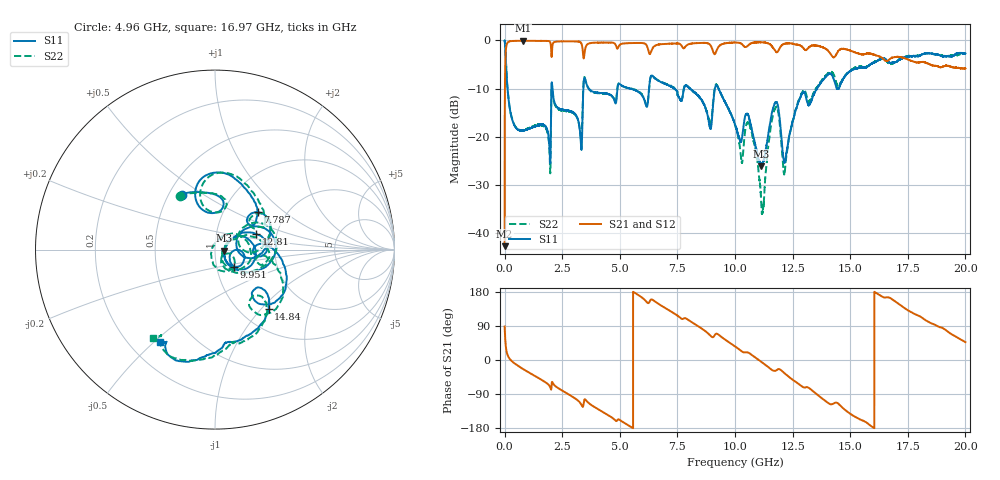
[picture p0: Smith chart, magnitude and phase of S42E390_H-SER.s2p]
! Created Wed Nov 25 22:14:23 2020
# khz S ma R 50
! 2 Port Network Data from SP1.SP block
! freq  magS11  angS11  magS21  angS21  magS12  angS12  magS22  angS22
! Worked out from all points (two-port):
!   20001 points, 300 kHz to 20 GHz, reference 50 ohm
!   highest |S21| = -0.07 dB at 794.3 MHz (marker M1); lowest = -42.8 dB at 300 kHz (marker M2)
!   |S21| within 3 dB of the highest: 40.74 MHz to 2.031 GHz (1.99 GHz wide, 192 % of centre); 3.459 GHz to 14.18 GHz (10.72 GHz wide, 122 % of centre)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
!   lowest |S11| = -26.2 dB at 11.15 GHz (marker M3), VSWR 1.10, Z = 55.1 - j0.678 ohm
!   |S11| at or under -10 dB: 126.5 MHz to 2.034 GHz (1.907 GHz wide, 177 % of centre); 2.075 GHz to 3.418 GHz (1.343 GHz wide, 48.9 % of centre); 9.28 GHz to 13.56 GHz (4.277 GHz wide, 37.5 % of centre)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
!   |S22| runs from -36.1 to 0.0 dB; largest |S21 - S12| = 0.016
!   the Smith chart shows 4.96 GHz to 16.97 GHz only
!   S11 on the Smith chart (normalised r, x): 4.96 GHz: 0.59, +0.41; 7.787 GHz: 1.44, +0.67; 9.951 GHz: 1.21, -0.24; 12.81 GHz: 1.57, +0.28; 14.84 GHz: 1.34, -1.10; 16.97 GHz: 0.33, -0.52
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300  0.9948 -0.3  0.007248 88.5  0.007244 89.5  0.993 -0.4
123300  0.3234 -75.8  0.9455 14.2  0.9454 14.2  0.3244 -75.9
794300  0.1155 -114.1  0.9918 -23.6  0.9902 -23.5  0.1168 -115.0
1911300  0.09897 -147.4  0.985 -65.4  0.9852 -65.4  0.094 -154.5
2121300  0.2507 -148.7  0.9472 -64.0  0.9477 -63.9  0.2455 -150.9
3334300  0.07255 -163.9  0.9276 -118.1  0.9282 -118.1  0.09135 -149.6
3512300  0.3819 173.8  0.8424 -105.0  0.8421 -105.1  0.384 179.3
4960300  0.3547 120.8  0.8754 -156.7  0.8756 -156.8  0.3577 123.2
6667300  0.3812 64.4  0.9059 148.6  0.9026 148.5  0.3838 57.2
7787300  0.3164 41.2  0.8302 110.0  0.8274 110.1  0.3217 38.8
9951300  0.1442 -42.2  0.9517 38.0  0.9527 37.9  0.1452 -55.4
1.00003e7  0.1339 -42.4  0.9515 35.9  0.9523 35.9  0.1327 -57.7
1.06533e7  0.1421 -42.0  0.9227 16.6  0.9246 16.6  0.1276 -70.7
1.11493e7  0.04896 -7.2  0.9548 -5.1  0.9557 -5.1  0.01829 -158.0
1.17133e7  0.2173 6.2  0.7992 -28.8  0.7996 -28.7  0.1897 9.9
1.21523e7  0.05389 -7.7  0.9251 -35.1  0.9249 -35.2  0.04178 -5.4
1.28093e7  0.2461 20.2  0.8927 -65.4  0.8912 -65.4  0.2504 13.3
1.33343e7  0.2427 6.8  0.8833 -79.7  0.8837 -79.6  0.253 -7.4
1.48403e7  0.4456 -47.8  0.8077 -134.8  0.8084 -135.0  0.4493 -49.7
1.66673e7  0.5936 -117.6  0.6263 165.3  0.614 165.4  0.5765 -121.9
1.69703e7  0.5969 -120.6  0.6718 153.8  0.6607 153.9  0.599 -125.1
2e7  0.7338 140.4  0.5087 47.0  0.5109 47.8  0.7307 137.5
